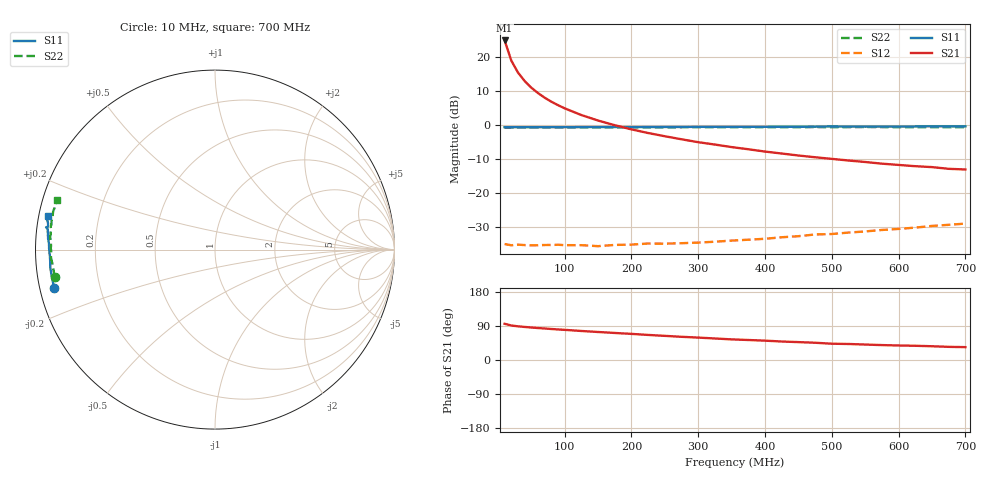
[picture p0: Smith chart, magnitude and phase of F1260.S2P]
! Date: Mon Aug 07 16:00:48 1995
# MHZ  S  MA  R  50.0000
!  POLYFET RF DEVICES
!  F1260
!  S PARAMETERS
!  VDS=12.5V, IDQ=800mA
!FREQ  S11MAG S11ANG S21MAG S21ANG S12MAG S12ANG S22MAG S22ANG
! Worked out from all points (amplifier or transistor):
!   34 points, 10 MHz to 700 MHz, reference 50 ohm
!   highest |S21| = 24.8 dB at 10 MHz (marker M1)
!   |S21| within 3 dB of that: start of sweep to 15.07 MHz
!   unconditionally stable (mu >= 1): 258.4 MHz to end of sweep
!   at 60 MHz: K = 0.23, MSG = 22.4 dB, |S12| = -35.4 dB
!   at 300 MHz: K = 1.06, MAG = 13.3 dB, |S12| = -34.6 dB
!   at 700 MHz: K = 1.34, MAG = 4.5 dB, |S12| = -29.1 dB
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10  0.9222 -166.7  17.4 95.6  0.01762 10.6  0.9056 -170.3
20  0.9233 -173.4  8.803 91.0  0.01691 6.1  0.9101 -175.3
30  0.9208 -175.7  5.873 88.9  0.01726 4.6  0.9148 -177.2
40  0.9204 -177.2  4.401 87.2  0.01702 4.5  0.9151 -178.4
50  0.9204 -177.9  3.515 85.7  0.01686 6.4  0.9131 -179.0
60  0.9215 -178.5  2.93 84.4  0.01693 4.5  0.9131 -179.7
70  0.9229 -178.8  2.504 83.1  0.01706 5.4  0.914 179.8
80  0.9227 -179.2  2.186 81.8  0.01708 5.4  0.916 179.6
90  0.9226 -179.6  1.944 80.6  0.01722 8.5  0.9145 179.2
100  0.9227 -179.9  1.746 79.5  0.01697 9.0  0.914 178.8
125  0.9247 179.5  1.391 76.6  0.01696 11.1  0.9146 178.0
150  0.9246 178.9  1.154 73.9  0.0164 13.5  0.9149 177.3
175  0.9251 178.5  0.9859 71.3  0.01711 14.9  0.9176 176.7
200  0.925 178.0  0.8562 68.9  0.01728 19.7  0.92 176.0
225  0.9268 177.6  0.7565 66.1  0.01794 21.4  0.9216 175.3
250  0.9284 177.1  0.6785 63.7  0.01785 24.7  0.9185 174.8
300  0.9321 176.3  0.5547 59.1  0.01852 29.2  0.9251 173.3
375  0.9349 175.1  0.4368 52.8  0.02041 34.5  0.9224 171.4
475  0.9391 173.1  0.333 45.5  0.02436 43.8  0.926 168.8
500  0.9494 172.5  0.3155 43.0  0.02475 46.2  0.9243 168.0
600  0.9417 171.0  0.2568 38.3  0.02942 48.7  0.9234 165.4
700  0.9488 168.6  0.2202 33.9  0.03523 52.4  0.9222 162.5
